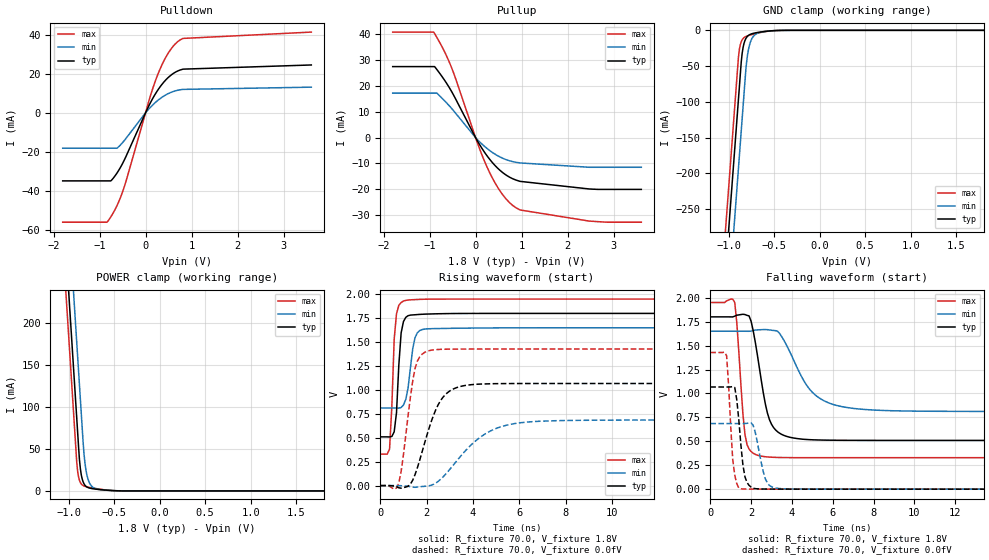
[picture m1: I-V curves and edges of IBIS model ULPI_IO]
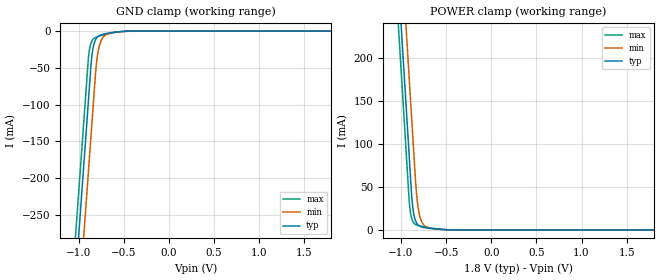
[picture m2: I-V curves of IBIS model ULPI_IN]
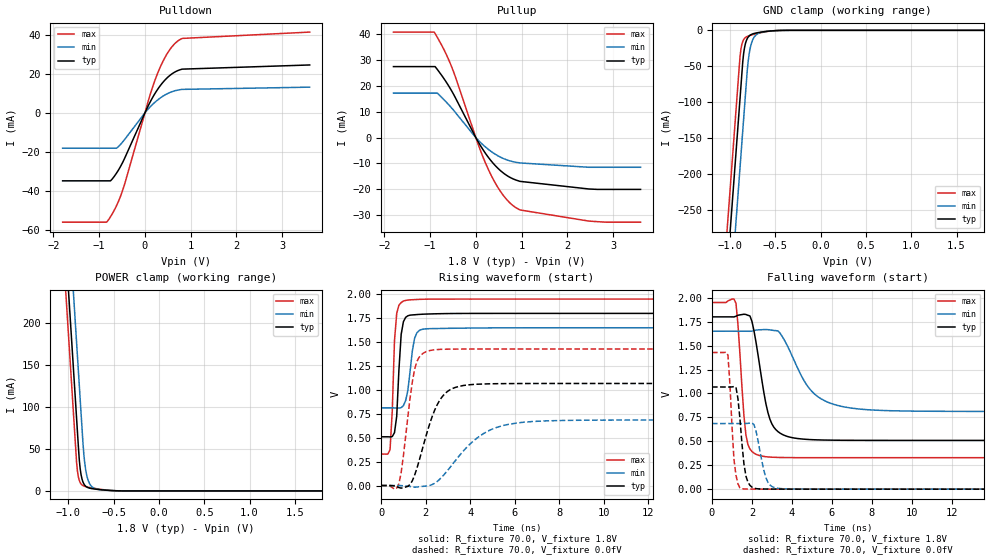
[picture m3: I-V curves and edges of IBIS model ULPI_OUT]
[IBIS Ver]   3.2
[File Name]   stulpi01.ibs
[File Rev]   1.0
[Date]   March 27th, 2007
[Notes]   These IBIS models are the proprietary information of
   STMicroelectronics and are disclosed to users solely for
   modeling and simulation purposes. STMicroelectronics reserves
   the right to change the IBIS models at any time and without
   notice.
[Copyright]   (c) STMicroelectronics
   All rights reserved. Reproduction in whole or part is prohibited
   without the written consent of the copyright holder.
[Component]   STULPI01
[Manufacturer] STMicroelectronics
[Package]
|   typ   min   max
R_pkg   0.1   NA   NA
L_pkg   1nH   NA   NA
C_pkg   100fF   NA   NA
[Pin] signal_name   model_name   R_pin   L_pin   C_pin
D1   DP   TRANSCEIVER_USB2   1.2378E-01   0.728nH  143.15fF
C1   DN   TRANSCEIVER_USB2   1.2419E-01   0.784nH  143.53fF
D3   ID   NC
F4   VBUS   NC
F1   CAP1   NC
F2   CAP2   NC
F5   XI   NC
F6   XO   NC
C2   RREF   NC
C3   PWRDWN   NC
A4   CLK   ULPI_IO   1.1592E-01   0.545nH   85.28fF
B1   D0   ULPI_IO   1.6911E-01   1.087nH  163.19fF
A1   D1   ULPI_IO   1.4149E-01   0.858nH  145.94fF
A2   D2   ULPI_IO   1.3482E-01   0.893nH  112.70fF
A3   D3   ULPI_IO   1.2080E-01   0.626nH   97.08fF
A5   D4   ULPI_IO   1.2203E-01   0.579nH  114.42fF
A6   D5   ULPI_IO   1.3109E-01   0.789nH  111.33fF
B6   D6   ULPI_IO   1.0111E-01   0.572nH  103.92fF
C6   D7   ULPI_IO   1.0677E-01   0.552nH  120.61fF
D6   STP   ULPI_IN   1.1349E-01   0.553nH  152.50fF
D5   NXT   ULPI_OUT   1.3754E-01   0.699nH  150.19fF
E5   DIR   ULPI_OUT   1.5162E-01   0.990nH  152.58fF
E2   VB_REF_FAULT  NC
D4   PSWn   NC
C4   RESETn   NC
F3   VBAT   POWER
E3   3V3V   POWER
E6   1V2V   POWER
B2   1V8VIO   POWER
B3   1V8VIO   POWER
B5   1V8VIO   POWER
C5   GND1   GND
D2   GND2   GND
B4   GND3   GND
E4   GND4   GND
E1   CPGND   GND
[Diff Pin]  inv_pin  vdiff  tdelay_typ tdelay_min tdelay_max
   D1   C1   NA   0   0   0
| Models and submodels in the file (4): ULPI_IO (I/O), ULPI_IN (Input), ULPI_OUT (Output), TRANSCEIVER_USB2 (Output)
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[Model]   ULPI_IO
Model_type   I/O
C_comp   1.4647pF  1.42605pF  1.53705pF
Vinl   =  800mV
Vinh   =  2.0V
Vmeas   =  900mV
Cref   =  62.5pF
Rref   =  1.0MOhm
Vref   =  900.0mV
[Model Spec]
Vinh 1.0204V 935.4mV 1.0744V
Vinl 706.6mV 650.6mV 761.6mV
[Temperature Range]   25.0  125.0   -40.0
[Voltage Range]   1.8V   1.65V   1.95V
[POWER Clamp Reference] 1.8V   1.65V   1.95V
[GND Clamp Reference]   0.0fV  0.0fV   0.0fV
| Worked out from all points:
|   slope of the pulldown table from 0 to 0.27 V, typ, clamps not added: 22.9 ohm
|   slope of the pullup table from 0 to 0.27 V, typ, clamps not added: 35.8 ohm
|   GND clamp passes 1 mA (typ) near -0.56 V on its own axis
|   POWER clamp passes 1 mA (typ) near -0.60 V on its own axis
|   rising waveform, R_fixture 70.0, V_fixture 1.8V: 20-80 % time 183ps typ, 280ps min, 176ps max; typ from 0.509 V to 1.8 V
|   falling waveform, R_fixture 70.0, V_fixture 1.8V: 20-80 % time 639ps typ, 1.38ns min, 325ps max; typ from 1.8 V to 0.509 V
|   rising waveform, R_fixture 70.0, V_fixture 0.0fV: 20-80 % time 884ps typ, 1.7ns min, 459ps max; typ from 0 V to 1.07 V
|   falling waveform, R_fixture 70.0, V_fixture 0.0fV: 20-80 % time 294ps typ, 411ps min, 234ps max; typ from 1.07 V to 0 V
[POWER Clamp]
-1.8V     1.6A       1.69A      1.547A
-1.12V    444.1mA    534.4mA    391.5mA
-910mV    87.15mA    177.4mA    34.49mA
-900mV    70.15mA    160.4mA    23.47mA
-880mV    37.31mA    126.4mA    12.56mA
-860mV    19.25mA    92.36mA    8.283mA
-840mV    10.84mA    58.36mA    6.441mA
-820mV    6.829mA    33.69mA    5.493mA
-790mV    4.236mA    15.37mA    4.629mA
-750mV    2.919mA    6.112mA    3.77mA
-680mV    1.858mA    2.004mA    2.5mA
1.8V      0A         0A         0A
[GND Clamp]
-1.8V     -1.642A    -1.738A    -1.583A
-900mV    -111.7mA   -208.1mA   -52.69mA
-880mV    -77.7mA    -174.1mA   -26.12mA
-860mV    -43.7mA    -140.1mA   -15.73mA
-840mV    -23.89mA   -106.1mA   -11.39mA
-820mV    -14.33mA   -72.07mA   -9.316mA
-810mV    -11.54mA   -55.34mA   -8.648mA
-790mV    -8.096mA   -33.26mA   -7.642mA
-760mV    -5.573mA   -16.46mA   -6.485mA
-710mV    -3.704mA   -6.229mA   -4.849mA
-640mV    -2.195mA   -2.406mA   -2.872mA
1.8V      402.7pA    17.66nA    51.86pA
| variable   typ   min   max
[Pullup Reference] 1.8V 1.65V 1.95V
| variable   typ   min   max
[Pulldown Reference] 0.0fV 0.0fV 0.0fV
[Pullup]
-1.8V     27.5mA     17.24mA    40.86mA
-910mV    27.5mA     17.24mA    40.86mA
-840mV    26.35mA    17.24mA    38.77mA
-670mV    22.13mA    14.2mA     33.09mA
-520mV    17.82mA    11.29mA    27.02mA
40mV      -1.264mA   -756uA     -2.036mA
260mV     -7.299mA   -4.35mA    -11.8mA
530mV     -12.65mA   -7.482mA   -20.61mA
820mV     -16.02mA   -9.339mA   -26.42mA
964mV     -16.93mA   -9.793mA   -27.99mA
2.47V     -19.88mA   -11.47mA   -32.31mA
3.6V      -20.04mA   -11.47mA   -32.73mA
[Pulldown]
-1.8V     -34.89mA   -18.17mA   -56.05mA
-840mV    -34.89mA   -18.17mA   -56.05mA
-760mV    -34.89mA   -18.17mA   -53.51mA
-620mV    -30.83mA   -18.14mA   -47.5mA
-470mV    -24.57mA   -14.44mA   -38.43mA
80mV      3.978mA    2.175mA    6.729mA
250mV     11.06mA    6.036mA    18.66mA
360mV     14.67mA    7.997mA    24.77mA
480mV     17.8mA     9.669mA    30.09mA
710mV     21.53mA    11.59mA    36.64mA
812mV     22.35mA    11.98mA    38.08mA
3.6V      24.49mA    13.12mA    41.33mA
[Ramp]
dV/dt_r 640.42664mV/881.11507ps 411.38247mV/1.69822ns 856.74423mV/452.97732ps
dV/dt_f 774.36724mV/635.17005ps 503.05951mV/1.38126ns 972.72878mV/315.86638ps
R_load = 70.0
[Rising Waveform]
R_fixture   = 70.0
V_fixture   = 1.8V
V_fixture_min = 1.65V
V_fixture_max = 1.95V
0s        509.5mV    811.7mV    328.8mV
400ps     508.5mV    811.7mV    381.1mV
500ps     513.7mV    811.8mV    831mV
600ps     562.5mV    811.5mV    1.529V
700ps     761mV      810.5mV    1.797V
900ps     1.596V     816.4mV    1.914V
1.1ns     1.759V     901mV      1.937V
1.5ns     1.786V     1.547V     1.945V
1.9ns     1.792V     1.636V     1.948V
24.9ns    1.8V       1.65V      1.95V
[Falling Waveform]
R_fixture   = 70.0
V_fixture   = 1.8V
V_fixture_min = 1.65V
V_fixture_max = 1.95V
0s        1.8V       1.65V      1.95V
1.2ns     1.808V     1.65V      1.951V
1.7ns     1.824V     1.65V      570.7mV
2ns       1.755V     1.652V     393.2mV
2.3ns     1.413V     1.664V     355.4mV
2.9ns     726.1mV    1.664V     335.1mV
4ns       537.7mV    1.388V     329.4mV
5.1ns     515.1mV    992.4mV    329mV
7ns       510.2mV    844.1mV    328.9mV
24.9ns    509.5mV    811.7mV    328.8mV
[Rising Waveform]
R_fixture   = 70.0
V_fixture   = 0.0fV
V_fixture_min = 0.0fV
V_fixture_max = 0.0fV
0s        0V         0V         0V
800ps     -23.07mV   -101uV     26.09mV
1.2ns     -6.811mV   -7.217mV   732mV
1.5ns     115.1mV    -17.67mV   1.224V
2.1ns     596.1mV    -1.912mV   1.41V
2.6ns     888.2mV    65.27mV    1.424V
3.1ns     1.004V     199.3mV    1.427V
4.5ns     1.063V     536.3mV    1.428V
6.1ns     1.067V     658.5mV    1.428V
24.8ns    1.067V     685.6mV    1.428V
[Falling Waveform]
R_fixture   = 70.0
V_fixture   = 0.0fV
V_fixture_min = 0.0fV
V_fixture_max = 0.0fV
0s        1.067V     685.6mV    1.428V
800ps     1.067V     685.7mV    1.395V
1.1ns     1.072V     685.4mV    308.9mV
1.3ns     931.6mV    685.4mV    56.95mV
1.5ns     462.5mV    685.4mV    3.614mV
1.9ns     39.83mV    691.4mV    1.068mV
2.2ns     5.634mV    597.9mV    580.9uV
2.7ns     1.432mV    108mV      200.5uV
3.3ns     642.4uV    8.858mV    57.96uV
24.9ns    0V         0V         0V
[Model]   ULPI_IN
Model_type   Input
C_comp   1.4654pF  1.42645pF  1.5376pF
Vinl = 800.0mV
Vinh = 2.0V
[Model Spec]
Vinh 1.0204V 935.4mV 1.0744V
Vinl 706.6mV 650.6mV 761.6mV
| variable   typ   min   max
[Temperature Range] 25.0 125.0 -40.0
| variable   typ   min   max
[Voltage Range] 1.8V 1.65V 1.95V
| variable   typ   min   max
[POWER Clamp Reference] 1.8V 1.65V 1.95V
| variable   typ   min   max
[GND Clamp Reference] 0.0fV 0.0fV 0.0fV
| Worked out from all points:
|   GND clamp passes 1 mA (typ) near -0.56 V on its own axis
|   POWER clamp passes 1 mA (typ) near -0.60 V on its own axis
[POWER Clamp]
-1.8V     1.6A       1.69A      1.548A
-1.12V    444.3mA    534.5mA    391.6mA
-910mV    87.28mA    177.5mA    34.59mA
-900mV    70.28mA    160.5mA    23.55mA
-880mV    37.42mA    126.5mA    12.61mA
-860mV    19.32mA    92.5mA     8.317mA
-840mV    10.88mA    58.5mA     6.467mA
-820mV    6.861mA    33.8mA     5.515mA
-790mV    4.254mA    15.44mA    4.647mA
-750mV    2.93mA     6.145mA    3.784mA
-680mV    1.865mA    2.014mA    2.509mA
1.8V      0A         0A         0A
[GND Clamp]
-1.8V     -1.642A    -1.738A    -1.583A
-900mV    -111.7mA   -208.1mA   -52.67mA
-880mV    -77.69mA   -174.1mA   -26.11mA
-860mV    -43.69mA   -140.1mA   -15.72mA
-840mV    -23.88mA   -106.1mA   -11.37mA
-820mV    -14.32mA   -72.05mA   -9.303mA
-810mV    -11.53mA   -55.32mA   -8.636mA
-790mV    -8.086mA   -33.24mA   -7.631mA
-760mV    -5.565mA   -16.45mA   -6.476mA
-710mV    -3.698mA   -6.221mA   -4.842mA
-640mV    -2.191mA   -2.402mA   -2.867mA
1.8V      400.6pA    17.63nA    49.91pA
[Model]   ULPI_OUT
Model_type Output
C_comp   1.40865pF  1.36735pF  1.47905pF
Vmeas = 900.0mV
Cref  = 62.5pF
Rref  = 1.0MOhm
Vref  = 900.0mV
[Temperature Range] 25.0 125.0 -40.0
[Voltage Range] 1.8V 1.65V 1.95V
[POWER Clamp Reference] 1.8V 1.65V 1.95V
[GND Clamp Reference] 0.0fV 0.0fV 0.0fV
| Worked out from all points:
|   slope of the pulldown table from 0 to 0.27 V, typ, clamps not added: 22.9 ohm
|   slope of the pullup table from 0 to 0.27 V, typ, clamps not added: 35.8 ohm
|   GND clamp passes 1 mA (typ) near -0.56 V on its own axis
|   POWER clamp passes 1 mA (typ) near -0.60 V on its own axis
|   rising waveform, R_fixture 70.0, V_fixture 1.8V: 20-80 % time 181ps typ, 273ps min, 170ps max; typ from 0.509 V to 1.8 V
|   falling waveform, R_fixture 70.0, V_fixture 1.8V: 20-80 % time 649ps typ, 1.41ns min, 326ps max; typ from 1.8 V to 0.509 V
|   rising waveform, R_fixture 70.0, V_fixture 0.0fV: 20-80 % time 890ps typ, 1.73ns min, 460ps max; typ from 0 V to 1.07 V
|   falling waveform, R_fixture 70.0, V_fixture 0.0fV: 20-80 % time 296ps typ, 414ps min, 232ps max; typ from 1.07 V to 0 V
[POWER Clamp]
-1.8V     1.6A       1.69A      1.547A
-1.12V    444.1mA    534.4mA    391.5mA
-910mV    87.15mA    177.4mA    34.49mA
-900mV    70.15mA    160.4mA    23.47mA
-880mV    37.31mA    126.4mA    12.56mA
-860mV    19.25mA    92.36mA    8.283mA
-840mV    10.84mA    58.36mA    6.441mA
-820mV    6.829mA    33.69mA    5.493mA
-790mV    4.236mA    15.37mA    4.629mA
-750mV    2.919mA    6.112mA    3.77mA
-680mV    1.858mA    2.004mA    2.5mA
1.8V      0A         0A         0A
[GND Clamp]
-1.8V     -1.641A    -1.738A    -1.582A
-900mV    -111.5mA   -207.8mA   -52.39mA
-880mV    -77.46mA   -173.8mA   -25.85mA
-860mV    -43.46mA   -139.8mA   -15.49mA
-840mV    -23.69mA   -105.8mA   -11.17mA
-820mV    -14.16mA   -71.82mA   -9.116mA
-810mV    -11.38mA   -55.1mA    -8.457mA
-790mV    -7.955mA   -33.06mA   -7.469mA
-760mV    -5.457mA   -16.31mA   -6.337mA
-710mV    -3.619mA   -6.137mA   -4.739mA
-640mV    -2.144mA   -2.357mA   -2.808mA
1.8V      390.8pA    17.3nA     46.34pA
| variable   typ   min   max
[Pullup Reference] 1.8V 1.65V 1.95V
| variable   typ   min   max
[Pulldown Reference] 0.0fV 0.0fV 0.0fV
[Pullup]
-1.8V     27.5mA     17.24mA    40.86mA
-910mV    27.5mA     17.24mA    40.86mA
-840mV    26.35mA    17.24mA    38.77mA
-670mV    22.13mA    14.2mA     33.09mA
-520mV    17.82mA    11.29mA    27.02mA
40mV      -1.264mA   -756uA     -2.036mA
260mV     -7.299mA   -4.35mA    -11.8mA
530mV     -12.65mA   -7.482mA   -20.61mA
820mV     -16.02mA   -9.339mA   -26.42mA
964mV     -16.93mA   -9.793mA   -27.99mA
2.47V     -19.88mA   -11.47mA   -32.31mA
3.6V      -20.04mA   -11.47mA   -32.73mA
[Pulldown]
-1.8V     -34.87mA   -18.17mA   -56.06mA
-840mV    -34.87mA   -18.17mA   -56.06mA
-760mV    -34.87mA   -18.17mA   -53.51mA
-620mV    -30.83mA   -18.14mA   -47.5mA
-470mV    -24.57mA   -14.44mA   -38.43mA
80mV      3.978mA    2.175mA    6.729mA
250mV     11.06mA    6.036mA    18.66mA
470mV     17.57mA    9.548mA    29.7mA
580mV     19.77mA    10.7mA     33.51mA
710mV     21.53mA    11.59mA    36.64mA
812mV     22.35mA    11.98mA    38.08mA
3.6V      24.49mA    13.12mA    41.33mA
[Ramp]
dV/dt_r 640.42663mV/886.36906ps 411.38229mV/1.72314ns 856.74406mV/454.33457ps
dV/dt_f 774.36714mV/644.07975ps 503.05902mV/1.40447ns 972.7288mV/316.46129ps
R_load = 70.0
[Rising Waveform]
R_fixture   = 70.0
V_fixture   = 1.8V
V_fixture_min = 1.65V
V_fixture_max = 1.95V
0s        509.5mV    811.7mV    328.8mV
400ps     508.5mV    811.7mV    373mV
500ps     511.9mV    811.8mV    780.3mV
600ps     553.1mV    811.6mV    1.517V
700ps     724.8mV    810.6mV    1.801V
900ps     1.581V     814.4mV    1.913V
1.1ns     1.759V     887.6mV    1.936V
1.5ns     1.786V     1.538V     1.944V
1.9ns     1.792V     1.636V     1.948V
24.9ns    1.8V       1.65V      1.95V
[Falling Waveform]
R_fixture   = 70.0
V_fixture   = 1.8V
V_fixture_min = 1.65V
V_fixture_max = 1.95V
0s        1.8V       1.65V      1.95V
1.2ns     1.807V     1.65V      1.943V
1.7ns     1.825V     1.65V      563.9mV
2ns       1.753V     1.651V     393.2mV
2.3ns     1.409V     1.664V     356.3mV
2.9ns     730.4mV    1.664V     335.3mV
4ns       538.8mV    1.397V     329.6mV
5.1ns     516.3mV    1V         329mV
7ns       510.4mV    846.2mV    328.9mV
24.9ns    509.5mV    811.7mV    328.8mV
[Rising Waveform]
R_fixture   = 70.0
V_fixture   = 0.0fV
V_fixture_min = 0.0fV
V_fixture_max = 0.0fV
0s        0V         0V         0V
800ps     -21.66mV   11.65uV    19.42mV
1.5ns     105.8mV    -17.77mV   1.213V
1.7ns     254mV      -13mV      1.339V
2.2ns     659.3mV    2.146mV    1.412V
2.7ns     915.6mV    82.29mV    1.424V
3.2ns     1.014V     221.1mV    1.427V
4.5ns     1.061V     528.9mV    1.428V
6.1ns     1.066V     653.6mV    1.428V
24.8ns    1.067V     685.6mV    1.428V
[Falling Waveform]
R_fixture   = 70.0
V_fixture   = 0.0fV
V_fixture_min = 0.0fV
V_fixture_max = 0.0fV
0s        1.067V     685.6mV    1.428V
800ps     1.067V     685.7mV    1.4V
1.1ns     1.072V     685.4mV    310.1mV
1.3ns     944.7mV    685.4mV    55.88mV
1.5ns     475.4mV    685.4mV    4.036mV
1.9ns     39.79mV    690.9mV    1.085mV
2.2ns     6.06mV     610.6mV    595.8uV
2.7ns     1.461mV    119.4mV    204.7uV
3.3ns     655.4uV    8.933mV    56.97uV
24.9ns    0V         0V         0V
